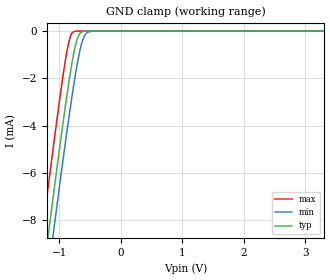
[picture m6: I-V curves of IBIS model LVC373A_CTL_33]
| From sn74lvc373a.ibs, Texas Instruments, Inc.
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[Model]   LVC373A_CTL_33
Model_type  Input
Vinl=0.8
Vinh=2.0
| variable   typ   min   max
C_comp   6.28pF   2.45pF   8.54pF
[Temperature Range]   40   100   -40
| Ambient temperature   25   85   -40
[Voltage range]   3.3   3   3.6
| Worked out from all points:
|   GND clamp passes 1 mA (typ) near -0.77 V on its own axis
[GND Clamp]
| LVC373A_CTL_33
|   Voltage   I(typ)   I(min)   I(max)
-5V       -90.43mA   -91.87mA   -88.61mA
-1.275V   -10.53mA   -12.13mA   -8.472mA
-1.18V    -8.586mA   -10.18mA   -6.518mA
-1.1V     -6.968mA   -8.566mA   -4.902mA
-885mV    -2.825mA   -4.363mA   -951.4uA
-825mV    -1.792mA   -3.264mA   -247.4uA
-765mV    -899.4uA   -2.23mA    -22.13uA
-700mV    -251.1uA   -1.236mA   -984.3nA
-635mV    -34.23uA   -487.3uA   -41.86nA
-585mV    -5.874uA   -166.8uA   -3.688nA
-510mV    -392.6nA   -20.95uA   -100.7pA
3.3V      9.4pA      17.51pA    8.777pA
